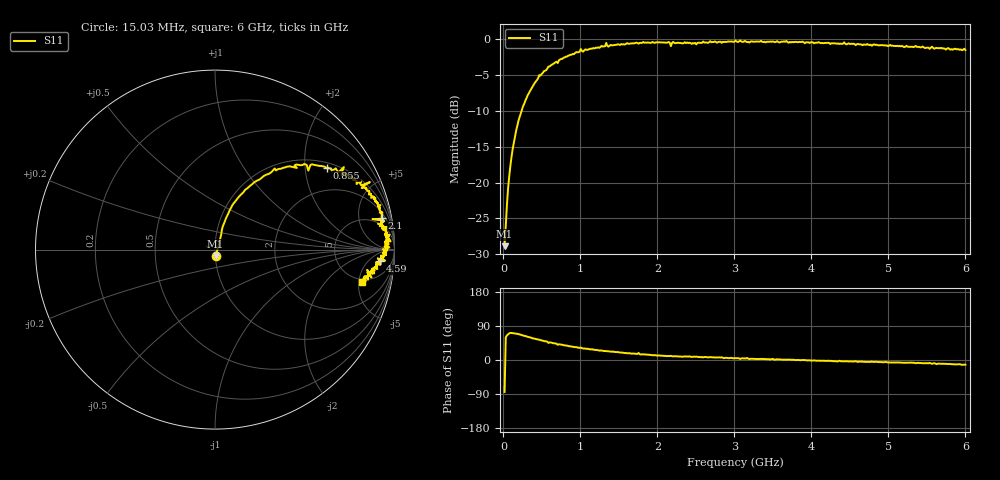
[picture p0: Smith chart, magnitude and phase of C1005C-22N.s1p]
!	Network	Analyzer	HP8753E.07.74:	Oct	30	2002	Serial	No.	JP38451487
!	Hewlett-Packard
!	7	Sep	2009	8:57:29
!	Frequency	S11
#	HZ	S	RI	R	50
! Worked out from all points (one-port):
!   400 points, 15.03 MHz to 6 GHz, reference 50 ohm
!   lowest |S11| = -28.9 dB at 15.03 MHz (marker M1), VSWR 1.07, Z = 50.2 - j3.6 ohm
!   |S11| at or under -10 dB: start of sweep to 236.2 MHz
!   S11 on the Smith chart (normalised r, x): 15.03 MHz: 1.00, -0.07; 855 MHz: 1.16, +2.60; 2.1 GHz: 3, +10; 4.59 GHz: 14, -12; 6 GHz: 4.52, -5.56
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1.502992e7  0.00356 -0.0358
3.002985e7  0.0256 0.0432
6.00297e7  0.0346 0.0842
9.002955e7  0.0416 0.124
1.95029e8  0.0989 0.251
3.150284e8  0.196 0.356
4.650277e8  0.333 0.452
7.650262e8  0.557 0.471
8.550257e8  0.622 0.455
1.320023e9  0.818 0.359
1.335023e9  0.863 0.376
1.365023e9  0.817 0.343
1.515022e9  0.857 0.307
1.725021e9  0.909 0.259
1.755021e9  0.881 0.297
1.785021e9  0.912 0.235
2.10002e9  0.929 0.178
2.145019e9  0.94 0.171
2.175019e9  0.877 0.17
2.205019e9  0.943 0.158
2.265019e9  0.931 0.158
2.505017e9  0.908 0.144
3.015015e9  0.973 0.0814
3.765011e9  0.952 0.0121
4.515007e9  0.927 -0.0561
4.590007e9  0.92 -0.0645
5.265004e9  0.878 -0.111
6e9  0.82 -0.181
